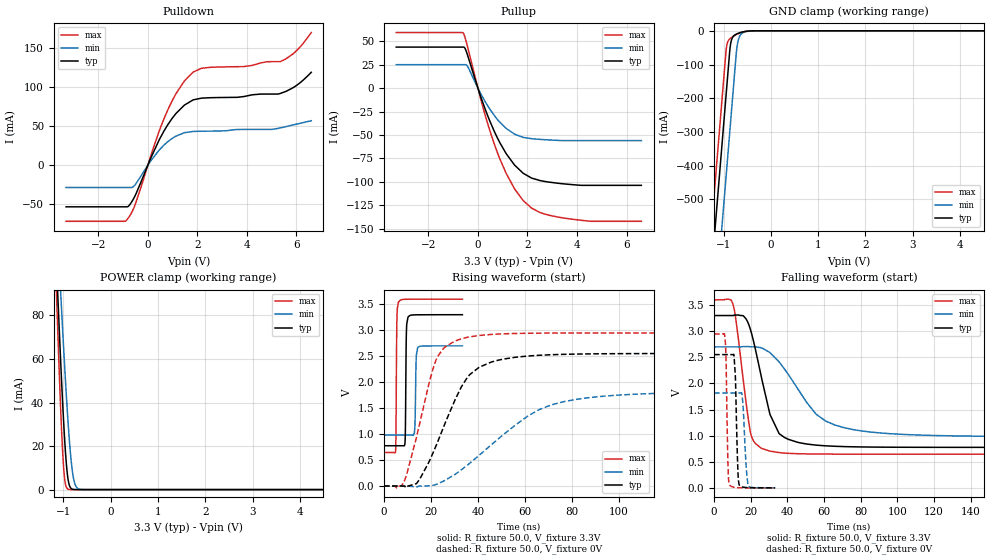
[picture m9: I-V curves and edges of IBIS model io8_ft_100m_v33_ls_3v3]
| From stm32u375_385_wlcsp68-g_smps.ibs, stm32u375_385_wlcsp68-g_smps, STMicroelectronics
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[Model]   io8_ft_100m_v33_ls_3v3
Model_type I/O
Polarity   Non-Inverting
Enable   Active-Low
| CAP_THRESHOLD on pad IOFT is "UDTCAPC" :
| Rising=30.0% of vddiom   Falling=70.0% of vddiom
| C_comp min and max val. don't necessarily correlate with the min and max pvt
| but are the smallest and greatest pad capacitance found.
| var   typ   min   max
C_comp   5.13864pF  4.98765pF  5.13964pF
|C_comp_pullup   3.32214pF  3.08522pF  3.41419pF
|C_comp_pulldown   1.81649pF  1.90243pF  1.72545pF
Vinl = 1.35V
Vinh = 1.8V
Vmeas = 1.65V   | Reference voltage for timing measurements
Cref  = 50.0pF   | Timing specification test load capacitance value
Rref  = 1.0MOhm   | Timing specification test load resistance value
Vref  = 1.815V   | Timing specification test load voltage
[Model Spec]
| TIME_THRESHOLD on pin ZIV33M is "CMOS" :
| Rising=50.0% of vddiom   Falling=50.0% of vddiom
Vinl 1.27350V 1.06350V 1.35850V
Vinh 1.78850V 1.51250V 1.89250V
| variable   typ   min   max
[Temperature Range] 25.0 130.0 -40.0
| variable   typ   min   max
[Voltage Range] 3.3V 2.7V 3.6V
| variable   typ   min   max
[POWER Clamp Reference] 3.3V 2.7V 3.6V
| variable   typ   min   max
[GND Clamp Reference] 0V 0V 0V
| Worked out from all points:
|   slope of the pulldown table from 0 to 0.495 V, typ, clamps not added: 14.3 ohm
|   slope of the pullup table from 0 to 0.495 V, typ, clamps not added: 13.8 ohm
|   GND clamp passes 1 mA (typ) near -0.50 V on its own axis
|   POWER clamp passes 1 mA (typ) near -0.85 V on its own axis
|   rising waveform, R_fixture 50.0, V_fixture 3.3V: 20-80 % time 304ps typ, 371ps min, 292ps max; typ from 0.776 V to 3.3 V
|   falling waveform, R_fixture 50.0, V_fixture 3.3V: 20-80 % time 10.6ns typ, 22.4ns min, 6.33ns max; typ from 3.3 V to 0.776 V
|   rising waveform, R_fixture 50.0, V_fixture 0V: 20-80 % time 15.2ns typ, 30.9ns min, 9.77ns max; typ from 0 V to 2.55 V
|   falling waveform, R_fixture 50.0, V_fixture 0V: 20-80 % time 1.11ns typ, 1.61ns min, 890ps max; typ from 2.55 V to 0 V
[POWER Clamp]
-3.3V     1.376A     1.183A     1.687A
-1.15V    107mA      132mA      94.23mA
-1.14V    101.7mA    127.5mA    87.74mA
-1.11V    86.11mA    114.3mA    68.77mA
-1.05V    56.42mA    88.49mA    34.19mA
-1V       34.12mA    67.92mA    12.34mA
-960mV    19.14mA    52.36mA    3.231mA
-900mV    4.863mA    31.3mA     221.9uA
-840mV    665uA      14.67mA    12.78uA
-790mV    105.7uA    5.908mA    1.173uA
-650mV    562.2nA    165.6uA    2.035nA
6.6V      0A         0A         0A
[GND Clamp]
-3.3V     -4.192A    -4.434A    -4.059A
-1.25V    -707.2mA   -948.8mA   -574.2mA
-950mV    -197.2mA   -438.8mA   -64.18mA
-940mV    -180.2mA   -421.8mA   -51.24mA
-870mV    -61.19mA   -302.8mA   -24.27mA
-850mV    -38.62mA   -268.8mA   -21.84mA
-800mV    -17.58mA   -183.8mA   -16.98mA
-730mV    -9.777mA   -65.72mA   -11.28mA
-710mV    -8.51mA    -43.04mA   -9.847mA
-620mV    -4.247mA   -8.765mA   -4.565mA
-390mV    -85.77uA   -309.6uA   -31.83uA
6.6V      2.503nA    356.6nA    1.779nA
| variable   typ   min   max
[Pullup Reference] 3.3V 2.7V 3.6V
| variable   typ   min   max
[Pulldown Reference] 0V 0V 0V
[Pullup]
-3.3V     43.84mA    25.07mA    59.35mA
-590mV    43.84mA    25.07mA    58.83mA
-520mV    42.41mA    25.07mA    54.03mA
-410mV    34.52mA    22.84mA    43.15mA
310mV     -23.64mA   -15.21mA   -30.46mA
880mV     -58mA      -36.24mA   -75.16mA
1.48V     -82.17mA   -49.14mA   -107.6mA
1.83V     -90.96mA   -52.61mA   -120.1mA
2.17V     -96.08mA   -54mA      -128.2mA
2.85V     -100.3mA   -55.28mA   -135.6mA
3.88V     -103.2mA   -56.04mA   -140.2mA
6.6V      -103.8mA   -56.04mA   -142.2mA
[Pulldown]
-3.3V     -53.27mA   -28.52mA   -71.84mA
-850mV    -53.27mA   -28.52mA   -70.02mA
-500mV    -38.18mA   -24.47mA   -49.51mA
460mV     32.61mA    19.53mA    43.99mA
800mV     51.7mA     30.09mA    70.55mA
1.14V     66.56mA    37.47mA    92mA
1.48V     77.24mA    41.82mA    108.3mA
1.83V     83.91mA    43.43mA    119.6mA
2.17V     86.16mA    43.73mA    124.5mA
5.35V     92.17mA    47.94mA    133mA
5.95V     101.3mA    52.36mA    145.4mA
6.6V      119.3mA    57.17mA    170.3mA
[Ramp]
dV/dt_r 1.53142V/15.05049ns 1.09004V/30.83024ns 1.76896V/9.63127ns
dV/dt_f 1.51461V/9.87606ns 1.03174V/21.995ns 1.77292V/6.28915ns
R_load = 50.0
| Removed startup time: 0s 0s 0s  .
| Removed end time: 33.4ns.
[Rising Waveform]
R_fixture   = 50.0
V_fixture   = 3.3V
V_fixture_min = 2.7V
V_fixture_max = 3.6V
0s        775.7mV    980.2mV    645.1mV
4.95ns    775.7mV    980.2mV    677.4mV
5.5ns     775.7mV    980.2mV    3.153V
6.15ns    775.7mV    980.2mV    3.54V
8.95ns    830mV      980.2mV    3.596V
9.55ns    2.949V     980.2mV    3.597V
10.25ns   3.254V     980.2mV    3.597V
12.95ns   3.296V     1.024V     3.599V
14.35ns   3.298V     2.666V     3.599V
33.4ns    3.3V       2.699V     3.6V
| Removed startup time: 0s 0s 0s  .
| Removed end time: 248.4ns.
[Falling Waveform]
R_fixture   = 50.0
V_fixture   = 3.3V
V_fixture_min = 2.7V
V_fixture_max = 3.6V
0s        3.3V       2.7V       3.6V
10.2ns    3.3V       2.7V       3.529V
16ns      3.295V     2.706V     2.048V
19.65ns   3.054V     2.702V     1.099V
26.3ns    2.045V     2.676V     751.9mV
30.5ns    1.408V     2.591V     703.8mV
35.5ns    1.039V     2.412V     675.7mV
55.65ns   818.6mV    1.412V     648.3mV
71ns      790.3mV    1.152V     645.9mV
248.4ns   775.7mV    980.4mV    645.1mV
| Removed startup time: 0s 0s 0s  .
| Removed end time: 248.4ns.
[Rising Waveform]
R_fixture   = 50.0
V_fixture   = 0V
V_fixture_min = 0V
V_fixture_max = 0V
0s        11.93nV    102.1nV    24.43nV
7.75ns    6.853uV    100.5nV    20.93mV
13.9ns    50.51mV    -17.31mV   947.4mV
22.55ns   816.4mV    35.86mV    2.467V
32.9ns    1.905V     310.1mV    2.835V
36.55ns   2.147V     439.7mV    2.873V
45.65ns   2.387V     792.1mV    2.92V
65.9ns    2.518V     1.468V     2.944V
81.15ns   2.541V     1.664V     2.947V
248.4ns   2.552V     1.817V     2.948V
| Removed startup time: 0s 0s 0s  .
| Removed end time: 33.35ns.
[Falling Waveform]
R_fixture   = 50.0
V_fixture   = 0V
V_fixture_min = 0V
V_fixture_max = 0V
0s        2.552V     1.817V     2.948V
6.15ns    2.552V     1.817V     2.791V
7.55ns    2.552V     1.817V     490.9mV
8.2ns     2.552V     1.817V     82.55mV
10.9ns    2.528V     1.817V     12.27mV
13ns      325.4mV    1.817V     2.456mV
13.65ns   60.75mV    1.817V     1.655mV
15.7ns    15.13mV    1.638V     697.1uV
18.4ns    4.75mV     82.62mV    382.1uV
33.35ns   256.5uV    848.1uV    137.1uV
